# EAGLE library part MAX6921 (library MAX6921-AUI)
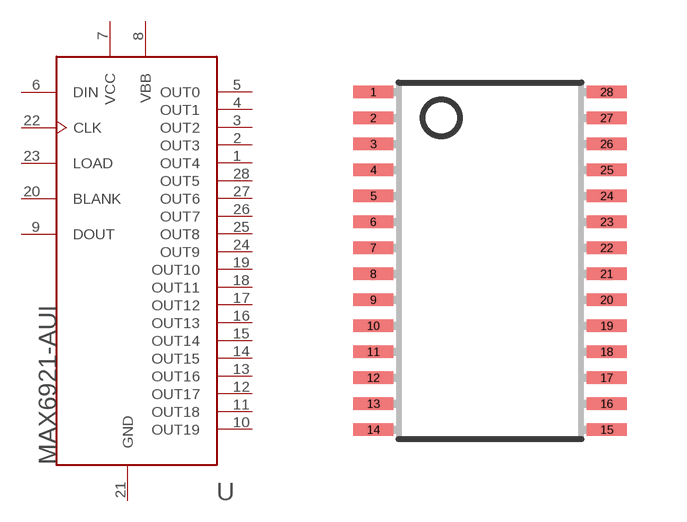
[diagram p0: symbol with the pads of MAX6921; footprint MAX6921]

Designator prefix -

## MAX6921  [MAX6921]
1  OUT4  out
2  OUT3  out
3  OUT2  out
4  OUT1  out
5  OUT0  out
6  DIN  in
7  VCC  pwr
8  VBB  sup
9  DOUT  out
10  OUT19  out
11  OUT18  out
12  OUT17  out
13  OUT16  out
14  OUT15  out
15  OUT14  out
16  OUT13  out
17  OUT12  out
18  OUT11  out
19  OUT10  out
20  BLANK  in
21  GND  sup
22  CLK  in
23  LOAD  in
24  OUT9  out
25  OUT8  out
26  OUT7  out
27  OUT6  out
28  OUT5  out

## Footprint MAX6921 (pad centres in mm)
smd 0.991 x 0.305: 1 -0.695,8.67; 2 -0.695,8.02; 3 -0.695,7.37; 4 -0.695,6.72; 5 -0.695,6.07; 6 -0.695,5.42; 7 -0.695,4.77; 8 -0.695,4.12; 9 -0.695,3.47; 10 -0.695,2.82; 11 -0.695,2.17; 12 -0.695,1.52; 13 -0.695,0.87; 14 -0.695,0.22; 15 5.14,0.22; 16 5.14,0.87; 17 5.14,1.52; 18 5.14,2.17; 19 5.14,2.82; 20 5.14,3.47; 21 5.14,4.12; 22 5.14,4.77; 23 5.14,5.42; 24 5.14,6.07; 25 5.14,6.72; 26 5.14,7.37; 27 5.14,8.02; 28 5.14,8.67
